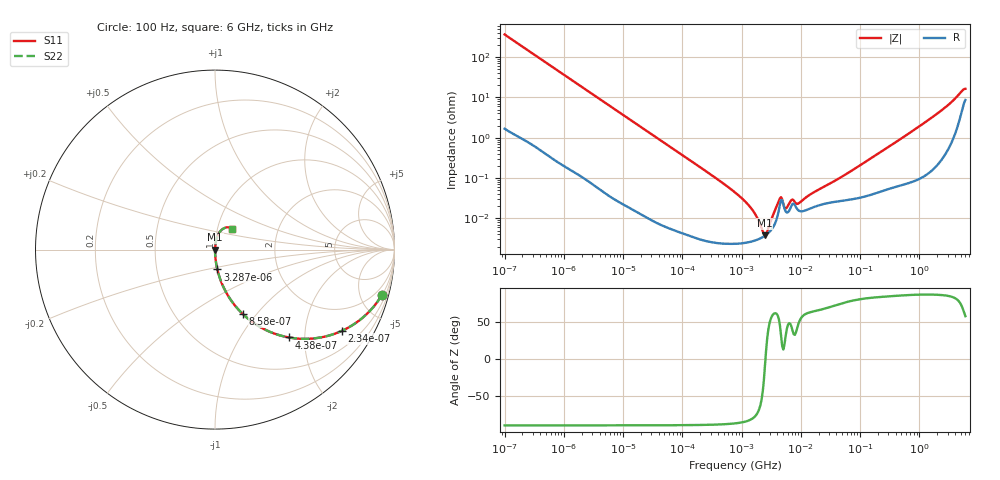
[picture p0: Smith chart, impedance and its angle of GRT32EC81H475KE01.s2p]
!Murata Part Number: GRT32EC81H475KE01
!These Parameters are Measured in Series Mode Connection
!Data Generated on Jun 19, 2026
!  o--ll--o
!Port1  Port2
!  o------o
!Operation Temp=25[degC], DC Bias Voltage=0[V]
!Freq. Start=100[Hz] Stop=6[GHz] 401[Steps]
# Hz S RI R 50
!Freq.(Hz) S11(Real) S11(Imag) S21(Real) S21(Imag) S12(Real) S12(Imag) S22(Real) S22(Imag)
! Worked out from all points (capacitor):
!   401 points, 100 Hz to 6 GHz, reference 50 ohm
!   read as one part in series: C = 4.37 uF near 109 Hz
!   lowest |Z| = 3.78 mohm at 2.481 MHz (marker M1)
!   series resonance near 2.53 MHz, so ESL is about 910 pH
!   S11 on the Smith chart (normalised r, x): 100 Hz: 1.03, -7.28; 234 Hz: 1.02, -3.12; 438 Hz: 1.01, -1.67; 858 Hz: 1.00, -0.85; 3.287 kHz: 1.00, -0.22; 6 GHz: 1.17, +0.28
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100  0.9287 -0.255  0.0713 0.255  0.0713 0.255  0.9287 -0.255
234  0.7072 -0.4525  0.2928 0.4525  0.2928 0.4525  0.7072 -0.4525
438  0.4108 -0.4893  0.5892 0.4893  0.5892 0.4893  0.4108 -0.4893
858  0.1556 -0.3598  0.8444 0.3598  0.8444 0.3598  0.1556 -0.3598
2008  0.0334 -0.1767  0.9666 0.1767  0.9666 0.1767  0.0334 -0.1767
3287  0.013 -0.1105  0.987 0.1105  0.987 0.1105  0.013 -0.1105
40335  0.000157 -0.0092  0.9998 0.0092  0.9998 0.0092  0.000157 -0.0092
774597  2.36e-05 -0.000441  1 0.000441  1 0.000441  2.36e-05 -0.000441
1267578  2.54e-05 -0.000225  1 0.000225  1 0.000225  2.54e-05 -0.000225
1896632  3.02e-05 -8.97e-05  1 8.97e-05  1 8.97e-05  3.02e-05 -8.97e-05
2481164  3.73e-05 -6.2e-06  1 6.2e-06  1 6.2e-06  3.73e-05 -6.2e-06
3245845  5.45e-05 8.66e-05  0.9999 -8.66e-05  0.9999 -8.66e-05  5.45e-05 8.66e-05
4440638  0.00022 0.000225  0.9998 -0.000225  0.9998 -0.000225  0.00022 0.000225
5809218  0.00014 0.000121  0.9999 -0.000121  0.9999 -0.000121  0.00014 0.000121
6948629  0.000205 0.000198  0.9998 -0.000198  0.9998 -0.000198  0.000205 0.000198
9090158  0.000158 0.000172  0.9998 -0.000172  0.9998 -0.000172  0.000158 0.000172
1.555665e7  0.000184 0.000378  0.9998 -0.000378  0.9998 -0.000378  0.000184 0.000378
5.449875e7  0.00028 0.00115  0.9997 -0.00115  0.9997 -0.00115  0.00028 0.00115
3.124326e8  0.00058 0.00609  0.9994 -0.00609  0.9994 -0.00609  0.00058 0.00609
1.95892e9  0.00348 0.0384  0.9965 -0.0384  0.9965 -0.0384  0.00348 0.0384
4.009986e9  0.0204 0.0895  0.9796 -0.0895  0.9796 -0.0895  0.0204 0.0895
6e9  0.0941 0.1154  0.9059 -0.1154  0.9059 -0.1154  0.0941 0.1154
